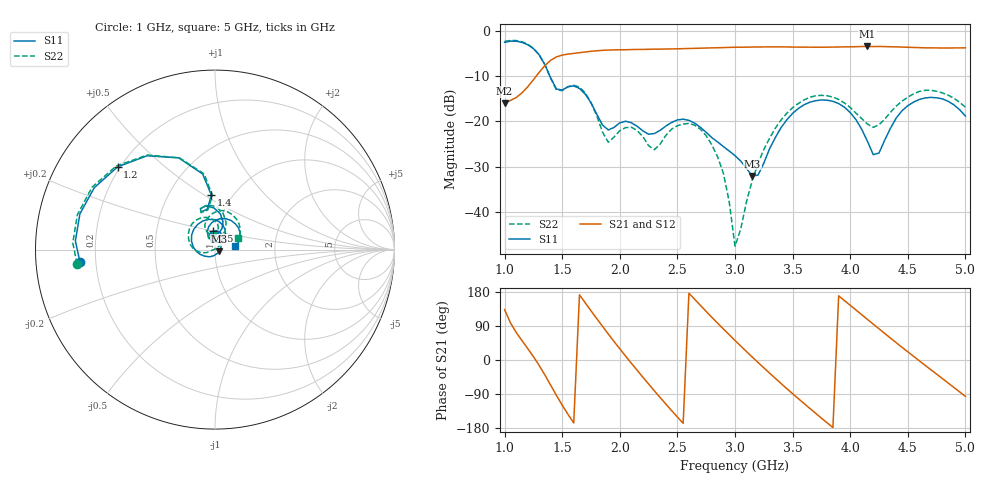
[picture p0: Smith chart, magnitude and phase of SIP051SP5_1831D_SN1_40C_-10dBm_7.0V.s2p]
# GHz  S  dB  R  50
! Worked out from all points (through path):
!   81 points, 1 GHz to 5 GHz, reference 50 ohm
!   highest |S21| = -3.35 dB at 4.15 GHz (marker M1); lowest = -15.9 dB at 1 GHz (marker M2)
!   lowest |S11| = -32.1 dB at 3.15 GHz (marker M3), VSWR 1.05, Z = 52.3 - j1.06 ohm
!   |S11| at or under -10 dB: 1.394 GHz to end of sweep
!   |S22| runs from -47.7 to -2.0 dB; largest |S21 - S12| = 0.0027
!   S11 on the Smith chart (normalised r, x): 1 GHz: 0.14, -0.05; 1.2 GHz: 0.19, +0.36; 1.4 GHz: 0.80, +0.54; 2.5 GHz: 0.96, +0.20; 5 GHz: 1.25, +0.05
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1  -2.44 -174.7  -15.95 132.9  -15.95 132.8  -2.24 -174.0
1.2  -2.95 139.7  -12.33 30.5  -12.31 30.6  -2.84 139.8
1.4  -10.34 93.8  -6.42 -66.5  -6.41 -66.6  -10.43 92.6
1.55  -12.29 109.6  -5.05 -143.3  -5.04 -143.3  -12.28 109.2
1.7  -13.92 81.5  -4.57 150.9  -4.58 150.7  -13.64 77.6
1.85  -20.79 78.6  -4.21 88.8  -4.20 88.7  -22.36 66.5
2.05  -19.94 99.9  -4.07 10.4  -4.08 10.3  -21.36 101.1
2.2  -22.07 92.1  -4.00 -45.4  -4.00 -45.3  -23.36 86.0
2.35  -21.97 107.5  -3.94 -98.9  -3.93 -98.9  -25.02 118.1
2.5  -19.66 95.6  -3.88 -150.4  -3.87 -150.4  -20.94 108.4
2.65  -20.36 70.1  -3.77 160.1  -3.77 160.0  -20.82 76.9
2.85  -24.56 50.0  -3.63 96.9  -3.62 96.8  -27.90 42.7
3  -27.59 35.6  -3.53 51.5  -3.52 51.5  -47.67 73.0
3.15  -32.09 -24.1  -3.47 7.6  -3.47 7.8  -33.01 -165.4
3.45  -19.61 -174.7  -3.45 -75.7  -3.46 -75.5  -18.16 176.3
3.7  -15.38 124.7  -3.52 -140.6  -3.52 -140.6  -14.30 131.0
3.9  -16.03 82.0  -3.47 169.2  -3.47 169.1  -15.11 97.7
4.15  -24.41 54.5  -3.35 107.0  -3.35 107.2  -20.58 86.9
4.25  -27.00 100.1  -3.35 82.4  -3.37 82.2  -20.73 109.0
4.35  -21.48 116.8  -3.41 57.7  -3.41 57.8  -17.95 115.6
4.65  -14.78 70.3  -3.65 -13.9  -3.64 -13.8  -13.08 78.9
5  -18.78 9.8  -3.65 -96.0  -3.65 -95.9  -16.82 25.4
